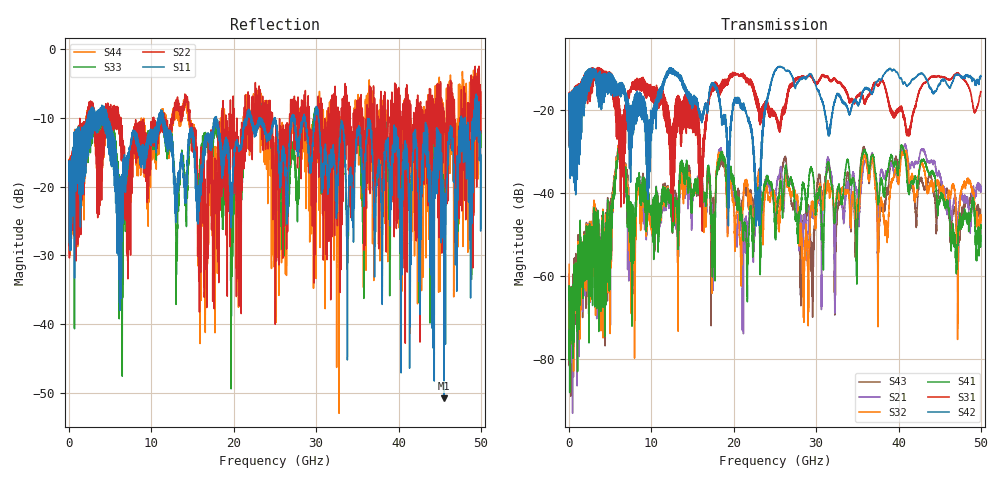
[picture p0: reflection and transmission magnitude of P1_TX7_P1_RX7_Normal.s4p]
!Keysight Technologies,N5225B,MY57041031,A.13.20.10
!Date: Friday, May 31, 2019 11:24:34
!Correction: S11(Full 4 Port(1,2,3,4))
!S12(Full 4 Port(1,2,3,4))
!S13(Full 4 Port(1,2,3,4))
!S14(Full 4 Port(1,2,3,4))
!S21(Full 4 Port(1,2,3,4))
!S22(Full 4 Port(1,2,3,4))
!S23(Full 4 Port(1,2,3,4))
!S24(Full 4 Port(1,2,3,4))
!S31(Full 4 Port(1,2,3,4))
!S32(Full 4 Port(1,2,3,4))
!S33(Full 4 Port(1,2,3,4))
!S34(Full 4 Port(1,2,3,4))
!S41(Full 4 Port(1,2,3,4))
!S42(Full 4 Port(1,2,3,4))
!S43(Full 4 Port(1,2,3,4))
!S44(Full 4 Port(1,2,3,4))
!S4P File: Measurements: <S11,S12,S13,S14>,
!<S21,S22,S23,S24>,
!<S31,S32,S33,S34>,
!<S41,S42,S43,S44>:
# Hz S  dB  R 50.0
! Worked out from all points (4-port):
!   5000 points, 10 MHz to 50 GHz, reference 50 ohm
!   strongest paths, dB at 10 MHz, 12.51 GHz, 25.01 GHz, 37.51 GHz, 50 GHz:
!     S42: -19.7, -10.0, -10.6, -12.9, -11.8
!     S31: -19.4, -39.5, -20.8, -14.0, -15.5
!     S41: -65.9, -49.0, -47.2, -42.2, -47.6
!     S32: -57.2, -42.9, -41.4, -72.2, -45.2
!     S21: -59.5, -43.5, -41.8, -55.2, -39.0
!     S43: -60.8, -48.3, -45.2, -46.8, -46.1
!   lowest |S11| = -50.8 dB at 45.52 GHz (marker M1), VSWR 1.01, Z = 50.2 + j0.175 ohm
!   |S11| at or under -10 dB: 4.613 GHz to 10.86 GHz (6.246 GHz wide, 80.7 % of centre); 11.46 GHz to 17.73 GHz (6.278 GHz wide, 43 % of centre); 30.28 GHz to 47.6 GHz (17.32 GHz wide, 44.5 % of centre)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
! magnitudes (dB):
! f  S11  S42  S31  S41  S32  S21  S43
! 10 MHz  -19.1  -19.7  -19.4  -65.9  -57.2  -59.5  -60.8
! 6.14 GHz  -24.9  -13.5  -32.0  -28.9  -28.4  -29.0  -28.5
! 7.8 GHz  -12.4  -17.8  -14.9  -43.9  -49.1  -45.6  -46.8
! 22.93 GHz  -10.6  -39.5  -17.3  -40.2  -37.0  -38.9  -37.2
! 25.41 GHz  -14.0  -9.5  -24.2  -41.1  -45.3  -35.9  -41.9
! 45.52 GHz  -50.8  -12.7  -12.0  -42.3  -40.0  -39.3  -39.9
! 50 GHz  -15.4  -11.8  -15.5  -47.6  -45.2  -39.0  -46.1
